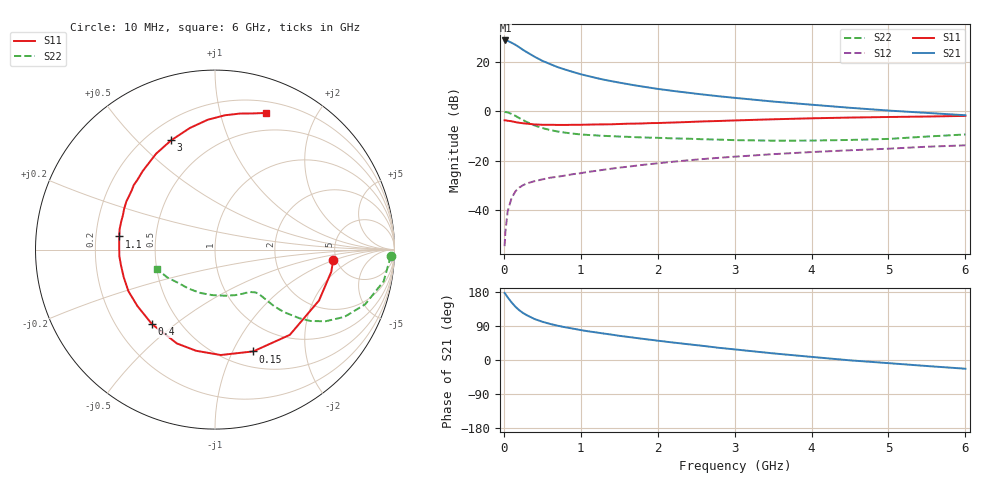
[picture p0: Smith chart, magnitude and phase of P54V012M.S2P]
! SIEMENS Small Signal Semiconductors
! BFP183
! Si NPN RF Bipolar Junction Transistor in SOT143
! VCE = 4 V  IC = 12 mA
! Common Emitter S-Parameters:  March  1996
# GHz  S  MA  R  50
!  f  S11  S21  S12  S22
! GHz  MAG  ANG  MAG  ANG  MAG  ANG  MAG  ANG
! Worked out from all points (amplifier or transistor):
!   36 points, 10 MHz to 6 GHz, reference 50 ohm
!   highest |S21| = 28.9 dB at 20 MHz (marker M1)
!   |S21| within 3 dB of that: start of sweep to 211 MHz
!   unconditionally stable (mu >= 1): 1.103 GHz to 5.59 GHz
!   at 250 MHz: K = 0.35, MSG = 27.6 dB, |S12| = -30.0 dB
!   at 1.4 GHz: K = 1.09, MAG = 16.0 dB, |S12| = -23.3 dB
!   at 6 GHz: K = 0.95, MSG = 6.1 dB, |S12| = -13.8 dB
!   S11 on the Smith chart (normalised r, x): 10 MHz: 4.69, -0.96; 150 MHz: 0.67, -1.21; 400 MHz: 0.35, -0.41; 1.1 GHz: 0.30, +0.06; 3 GHz: 0.30, +0.63; 6 GHz: 0.31, +1.39
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0.01  0.6609 -5.0  27.87 176.9  0.0018 82.5  0.9815 -2.1
0.02  0.6597 -10.7  27.93 174.3  0.0035 89.6  0.972 -4.2
0.05  0.6454 -26.0  27.38 165.3  0.0093 80.0  0.9562 -10.6
0.1  0.632 -48.7  25.13 152.2  0.0171 67.9  0.8907 -20.0
0.15  0.6059 -69.4  22.79 140.7  0.0235 61.1  0.8136 -27.4
0.2  0.5882 -86.9  20.33 131.4  0.0281 55.3  0.7348 -32.9
0.25  0.5735 -100.6  17.94 123.9  0.0315 51.5  0.6659 -36.7
0.3  0.5643 -112.1  16.08 118.1  0.0342 48.7  0.6067 -39.1
0.4  0.5437 -130.3  13.01 108.1  0.038 45.4  0.5183 -42.2
0.5  0.5346 -144.0  10.76 101.0  0.0413 43.1  0.4587 -43.7
0.6  0.5352 -154.4  9.253 95.3  0.0446 43.6  0.419 -44.2
0.7  0.5313 -163.3  7.984 90.5  0.0468 44.0  0.3899 -44.6
0.9  0.5342 -176.1  6.365 82.8  0.0528 44.7  0.353 -45.2
1.1  0.5388 172.2  5.245 75.6  0.0589 45.7  0.3314 -46.4
1.5  0.5547 155.9  3.867 63.9  0.0716 46.0  0.3082 -50.3
1.8  0.5693 144.6  3.219 56.0  0.0814 46.0  0.2954 -54.7
2.2  0.5946 132.7  2.62 46.1  0.0945 44.2  0.2828 -61.8
3  0.6559 111.9  1.893 28.0  0.1197 39.1  0.2602 -80.0
3.5  0.6918 101.7  1.591 17.5  0.1348 35.8  0.2541 -93.6
4.5  0.7504 85.8  1.187 -0.9  0.1618 28.0  0.2626 -124.1
5.5  0.7873 74.5  0.934 -15.9  0.1911 20.8  0.3079 -149.8
6  0.8116 69.7  0.837 -23.0  0.204 16.5  0.34 -161.2
